ORGANIZATION_BLOCK OB 1
BEGIN

	// Start timer and let it expire
	__STWRST
	L		0
	SI		T 10
	SET
	R		T 10
	U		T 10
	__ASSERT==	__STW VKE,	0
	SET
	L		W#16#0010
	SI		T 10
	U		T 10
	__ASSERT==	__STW VKE,	1
	L		T 10
	__ASSERT>=	__ACCU 1,	5
	__SLEEP		101
	U		T 10
	__ASSERT==	__STW VKE,	0
	L		T 10
	__ASSERT==	__ACCU 1,	0


	// Start timer and reset VKE before it expires
	__STWRST
	L		0
	SI		T 10
	SET
	R		T 10
	U		T 10
	__ASSERT==	__STW VKE,	0
	SET
	L		W#16#0010
	SI		T 10
	U		T 10
	__ASSERT==	__STW VKE,	1
	L		T 10
	__ASSERT>=	__ACCU 1,	5
	CLR
	L		W#16#0010
	SI		T 10
	U		T 10
	__ASSERT==	__STW VKE,	0
	L		T 10
	__ASSERT>=	__ACCU 1,	5
	__SLEEP		101
	U		T 10
	__ASSERT==	__STW VKE,	0
	L		T 10
	__ASSERT==	__ACCU 1,	__ACCU 2


	// Reset signal
	__STWRST
	L		0
	SI		T 10
	SET
	R		T 10
	U		T 10
	__ASSERT==	__STW VKE,	0
	SET
	L		W#16#0010
	SI		T 10
	U		T 10
	__ASSERT==	__STW VKE,	1
	L		T 10
	__ASSERT>=	__ACCU 1,	5
	SET
	R		T 10
	U		T 10
	__ASSERT==	__STW VKE,	0
	L		T 10
	__ASSERT==	__ACCU 1,	0
	__SLEEP		101
	U		T 10
	__ASSERT==	__STW VKE,	0
	L		T 10
	__ASSERT==	__ACCU 1,	0


	// Test LC
	__STWRST
	L		0
	SI		T 10
	SET
	R		T 10
	U		T 10
	__ASSERT==	__STW VKE,	0
	SET
	L		W#16#1010
	SI		T 10
	U		T 10
	__ASSERT==	__STW VKE,	1
	__SLEEP		101
	CLR
	L		W#16#1010
	SI		T 10
	U		T 10
	__ASSERT==	__STW VKE,	0
	L		T 10
	__ASSERT>	__ACCU 1,	0
	__ASSERT<	__ACCU 1,	10
	DTB
	XOW		W#16#1000
	__SLEEP		101
	LC		T 10
	__ASSERT==	__ACCU 1,	__ACCU 2


	// Test timer parameter
	AUF		DB 1
	L		DBW 0
	__ASSERT==	__ACCU 1,	24
	CALL FB 1, DB 1 (
		TIMER_VAR	:= T 42
	)


	CALL SFC 46 // STOP CPU
END_ORGANIZATION_BLOCK


FUNCTION_BLOCK FB 1
	VAR_INPUT
		TIMER_VAR	: TIMER
	END_VAR
BEGIN
	L		DIW 0
	__ASSERT==	__ACCU 1,	42
	L		#TIMER_VAR
	__ASSERT==	__ACCU 1,	0
	U		#TIMER_VAR
	__ASSERT==	__STW VKE,	0

	SET
	L		S5T#10s
	SI		T 42
	CLR
	U		T 42
	__ASSERT==	__STW VKE,	1
	CLR
	U		#TIMER_VAR
	__ASSERT==	__STW VKE,	1
	L		#TIMER_VAR
	__ASSERT<>	__ACCU 1,	0

	SI		#TIMER_VAR
END_FUNCTION_BLOCK


DATA_BLOCK DB 1
	FB 1
BEGIN
	TIMER_VAR	:= T 24
END_DATA_BLOCK
